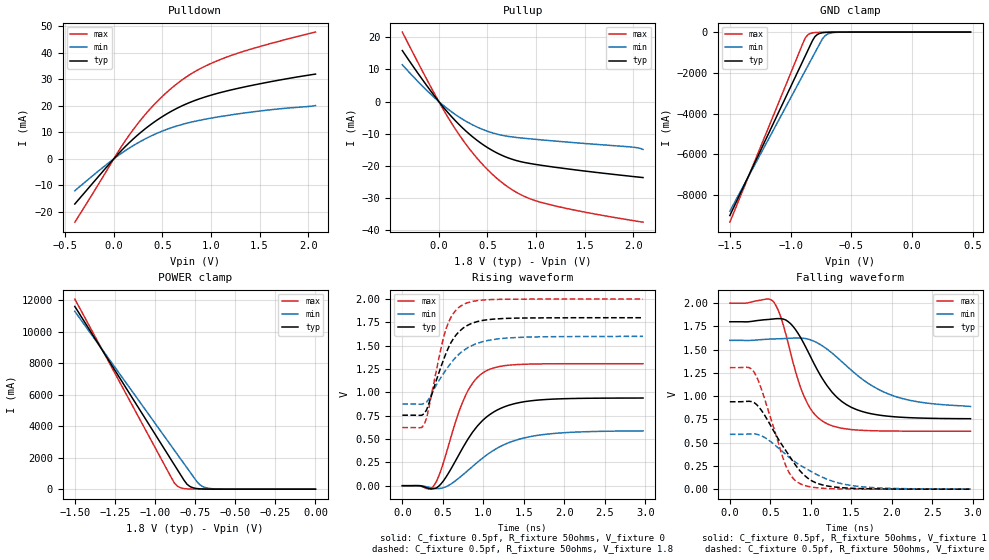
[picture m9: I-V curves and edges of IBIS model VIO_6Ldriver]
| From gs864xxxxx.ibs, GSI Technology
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|  signals   DQA1-DQA9, DQB1-DQB9, DQC1-DQC9, DQD1-DQD9
[Model]   VIO_6Ldriver
Model_type   I/O
Polarity   Non-Inverting
Vinl  =   0.54v
Vinh  =   1.08v
Vmeas =   0.9v
Cref  =   0pF
Rref  =   50
Vref  =   0.9v
|  variable   typ   min   max
C_comp   3.0pF   2.5pF   3.5pF
|  variable   typ   min   max
[Temperature Range]   50   0   100
|  variable   typ   min   max
[Voltage Range]   1.8   1.6   2.0
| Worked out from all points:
|   slope of the pulldown table from 0 to 0.27 V, typ, clamps not added: 27.7 ohm
|   slope of the pullup table from 0 to 0.27 V, typ, clamps not added: 30.3 ohm
|   GND clamp passes 1 mA (typ) near -0.58 V on its own axis
|   POWER clamp passes 1 mA (typ) near -0.61 V on its own axis
|   rising waveform, C_fixture 0.5pf, R_fixture 50ohms, V_fixture 0: 20-80 % time 457ps typ, 594ps min, 316ps max; typ from 0 V to 0.94 V
|   rising waveform, C_fixture 0.5pf, R_fixture 50ohms, V_fixture 1.8: 20-80 % time 285ps typ, 383ps min, 216ps max; typ from 0.756 V to 1.8 V
|   falling waveform, C_fixture 0.5pf, R_fixture 50ohms, V_fixture 1.8: 20-80 % time 452ps typ, 667ps min, 300ps max; typ from 1.8 V to 0.758 V
|   falling waveform, C_fixture 0.5pf, R_fixture 50ohms, V_fixture 0: 20-80 % time 416ps typ, 608ps min, 285ps max; typ from 0.94 V to 0 V
[Pulldown]
| voltage   typ   min   max
-400mV    -16.98mA   -11.99mA   -23.83mA
25mV      1.029mA    690uA      1.514mA
200mV     7.505mA    5.012mA    11.04mA
300mV     10.67mA    7.101mA    15.71mA
400mV     13.48mA    8.931mA    19.88mA
525mV     16.53mA    10.87mA    24.44mA
650mV     19.09mA    12.44mA    28.34mA
750mV     20.8mA     13.46mA    31mA
875mV     22.57mA    14.5mA     33.75mA
1.15V     25.51mA    16.29mA    38.24mA
1.525V    28.49mA    18.17mA    42.61mA
2.075V    31.98mA    20.13mA    47.82mA
[Pullup]
| voltage (VDDQ-Vout) typ   min   max
-375mV    15.82mA    11.4mA     21.57mA
-25mV     969.4uA    670.1uA    1.367mA
175mV     -6.111mA   -4.131mA   -8.754mA
300mV     -9.735mA   -6.479mA   -14.1mA
400mV     -12.2mA    -8.004mA   -17.84mA
525mV     -14.75mA   -9.477mA   -21.86mA
650mV     -16.72mA   -10.48mA   -25.17mA
850mV     -18.73mA   -11.33mA   -29.04mA
1.05V     -19.79mA   -11.9mA    -31.31mA
1.4V      -21.22mA   -12.79mA   -33.75mA
1.975V    -23.22mA   -14.11mA   -36.87mA
2.1V      -23.62mA   -14.88mA   -37.48mA
[GND Clamp]
| voltage   typ   min   max
-1.5V     -9.007A    -8.796A    -9.334A
-900mV    -1.426A    -2.122A    -562.9mA
-880mV    -1.174A    -1.9A      -292.9mA
-860mV    -921.1mA   -1.678A    -142.5mA
-820mV    -416.2mA   -1.233A    -38.58mA
-800mV    -222mA     -1.011A    -23.51mA
-780mV    -116.3mA   -788.8mA   -16.2mA
-740mV    -33.04mA   -348.7mA   -9.876mA
-720mV    -18.57mA   -198.2mA   -8.142mA
-700mV    -10.99mA   -111mA     -6.744mA
-660mV    -4.5mA     -34.67mA   -4.472mA
480mV     -45.44pA   551.3pA    -170.2pA
[POWER Clamp]
| voltage (VDDQ-Vout) typ   min   max
-1.5V     11.62A     11.31A     12.09A
-900mV    1.877A     2.768A     763.5mA
-880mV    1.553A     2.483A     398.4mA
-860mV    1.228A     2.198A     183.4mA
-840mV    903.6mA    1.913A     83.63mA
-800mV    304.2mA    1.344A     19.44mA
-780mV    154.7mA    1.059A     10.68mA
-740mV    39.51mA    489.9mA    4.639mA
-720mV    20.32mA    274.5mA    3.532mA
-680mV    5.894mA    82.85mA    2.298mA
-580mV    568.7uA    4.201mA    684.1uA
0V        586.7pA    1.815nA    370pA
[Ramp]
| voltage   typ   min   max
dV/dt_r   1.53/137p   1.35/170p   1.77/112p
dV/dt_f   1.51/136p   1.31/167p   1.77/112p
R_load  =   50ohms
[Rising Waveform]
C_fixture =   0.5pf
R_fixture =   50ohms
V_fixture =   0
| Time   V(typ)   V(min)   V(max)
0s        6.4nV      16.29nV    4.305nV
390ps     -31.54mV   -28.43mV   2.297mV
510ps     54.94mV    -20.79mV   254.9mV
660ps     272mV      55.71mV    693mV
780ps     456.4mV    141.5mV    966.6mV
900ps     610.7mV    231mV      1.136V
1.02ns    722.3mV    315.7mV    1.224V
1.29ns    855mV      452.6mV    1.289V
1.65ns    915.5mV    536.6mV    1.305V
2.97ns    939.5mV    587.4mV    1.307V
[Rising Waveform]
C_fixture =   0.5pf
R_fixture =   50ohms
V_fixture =   1.8
V_fixture_min =   1.6
V_fixture_max =   2.0
| Time   V(typ)   V(min)   V(max)
0s        755.6mV    874.9mV    622.8mV
270ps     772mV      882.6mV    656.3mV
300ps     813.9mV    897.2mV    726mV
480ps     1.282V     1.165V     1.483V
540ps     1.421V     1.243V     1.682V
630ps     1.575V     1.347V     1.847V
780ps     1.706V     1.463V     1.953V
1.02ns    1.775V     1.55V      1.991V
1.32ns    1.794V     1.584V     1.998V
2.97ns    1.8V       1.6V       2V
[Falling Waveform]
C_fixture =   0.5pf
R_fixture =   50ohms
V_fixture =   1.8
V_fixture_min =   1.6
V_fixture_max =   2.0
| Time   V(typ)   V(min)   V(max)
0s        1.8V       1.6V       2V
540ps     1.83V      1.615V     2.015V
630ps     1.833V     1.618V     1.848V
720ps     1.801V     1.621V     1.568V
900ps     1.588V     1.623V     1.03V
1.02ns    1.382V     1.597V     832.8mV
1.2ns     1.112V     1.505V     703.2mV
1.5ns     879.6mV    1.278V     641mV
1.95ns    784.8mV    1.026V     625.2mV
2.97ns    757.5mV    889mV      623.1mV
[Falling Waveform]
C_fixture =   0.5pf
R_fixture =   50ohms
V_fixture =   0
| Time   V(typ)   V(min)   V(max)
0s        939.8mV    589.4mV    1.307V
240ps     944.9mV    593.6mV    1.307V
300ps     930.2mV    594.5mV    1.259V
420ps     808.6mV    560.2mV    996.6mV
690ps     415.1mV    373.8mV    252.3mV
780ps     296.9mV    309.3mV    116.8mV
870ps     192.6mV    255.9mV    57.81mV
1.11ns    53.88mV    141.4mV    12.01mV
1.53ns    8.763mV    35.64mV    958uV
2.97ns    37.26uV    698uV      153.7nV
